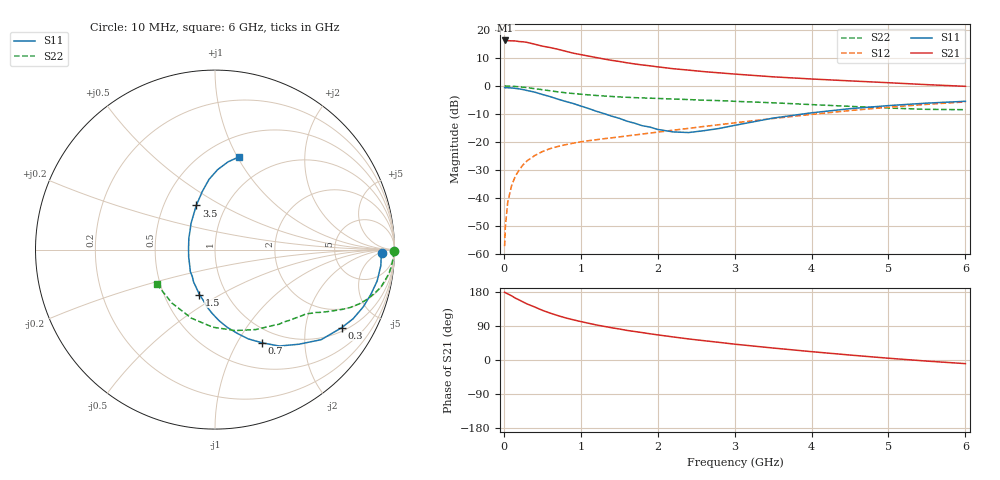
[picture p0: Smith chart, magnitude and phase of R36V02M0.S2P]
! SIEMENS Small Signal Semiconductors
! BFR181
! Si NPN RF Bipolar Junction Transistor in SOT23
! VCE = 6 V  IC = 2 mA
! Common Emitter S-Parameters:  May  1996
# GHz  S  MA  R  50
!  f  S11  S21  S12  S22
! GHz  MAG  ANG  MAG  ANG  MAG  ANG  MAG  ANG
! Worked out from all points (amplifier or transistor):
!   36 points, 10 MHz to 6 GHz, reference 50 ohm
!   highest |S21| = 16.2 dB at 20 MHz (marker M1)
!   |S21| within 3 dB of that: start of sweep to 679.9 MHz
!   unconditionally stable (mu >= 1): 1.626 GHz to 3.425 GHz
!   at 250 MHz: K = 0.23, MSG = 21.9 dB, |S12| = -28.1 dB
!   at 1.4 GHz: K = 0.94, MSG = 13.8 dB, |S12| = -18.5 dB
!   at 6 GHz: K = 0.86, MSG = 2.8 dB, |S12| = -5.7 dB
!   lowest NFmin = 1.35 dB at 450 MHz
!   S11 on the Smith chart (normalised r, x): 10 MHz: 27, -7; 300 MHz: 1.14, -3.16; 700 MHz: 0.81, -1.28; 1.5 GHz: 0.75, -0.40; 3.5 GHz: 0.73, +0.38; 6 GHz: 0.70, +1.01
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0.01  0.9325 -1.1  6.409 178.9  0.0014 97.2  0.9974 -0.6
0.02  0.9268 -2.0  6.449 177.5  0.0031 83.1  0.9961 -1.1
0.05  0.9283 -5.5  6.4 174.6  0.0084 88.1  0.9939 -2.6
0.1  0.9201 -11.0  6.345 169.5  0.0166 84.4  0.9879 -5.1
0.15  0.9036 -16.0  6.317 163.2  0.0248 80.2  0.9782 -7.8
0.3  0.8292 -31.6  5.966 148.1  0.0461 71.6  0.9321 -14.3
0.4  0.776 -40.3  5.533 140.0  0.0574 67.1  0.8934 -18.0
0.5  0.7049 -48.4  5.113 131.2  0.0676 63.6  0.8571 -20.7
0.6  0.6458 -56.3  4.827 123.9  0.0763 60.3  0.8195 -23.2
0.7  0.5827 -63.1  4.502 117.3  0.0833 58.6  0.7846 -25.1
0.8  0.5306 -69.6  4.153 111.3  0.0896 56.2  0.7556 -26.6
0.9  0.487 -74.6  3.837 106.2  0.0954 55.4  0.7325 -27.9
1.1  0.3962 -86.8  3.401 97.0  0.1057 53.8  0.693 -30.2
1.3  0.3221 -98.0  3.019 88.9  0.1148 53.5  0.6611 -32.0
1.5  0.2649 -109.2  2.726 81.9  0.1235 53.9  0.6374 -33.9
1.9  0.1848 -138.0  2.277 69.2  0.1447 54.8  0.6045 -37.8
2.2  0.1518 -165.4  2.025 60.9  0.1626 55.6  0.5835 -41.2
2.8  0.1748 142.6  1.709 46.5  0.204 55.6  0.5473 -49.5
3.5  0.2672 113.0  1.451 31.6  0.2628 53.1  0.5004 -62.9
4.5  0.3932 94.8  1.229 13.1  0.364 45.3  0.4326 -91.6
5.5  0.4938 81.6  1.053 -2.9  0.4701 33.2  0.3825 -128.9
6  0.5323 75.7  0.983 -9.6  0.5189 26.0  0.3771 -149.4
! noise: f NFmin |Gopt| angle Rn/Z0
0.45  1.35  0.6  17  0.4
0.9  1.45  0.5  36  0.4
1.8  1.8  0.31  80  0.37
